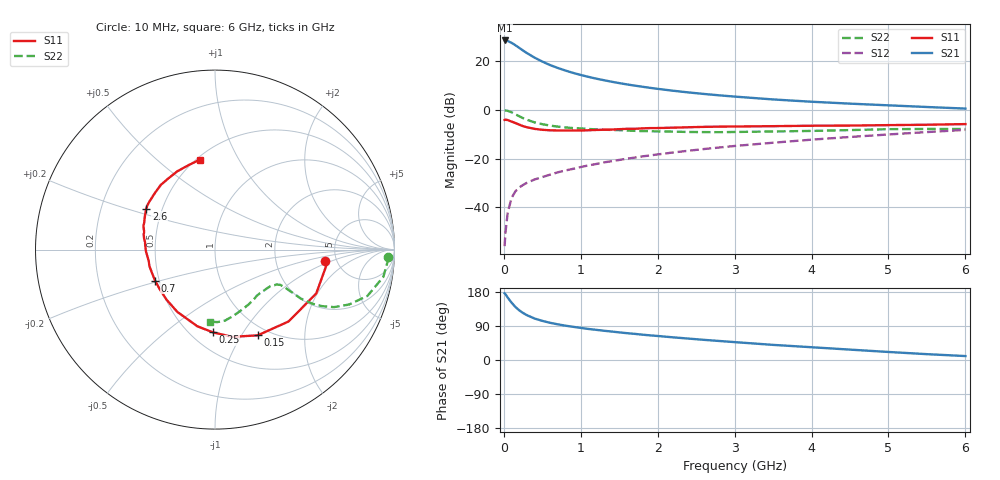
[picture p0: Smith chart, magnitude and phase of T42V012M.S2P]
! Infineon Technologies  Discrete & RF Semiconductors
! BFR182T
! Si NPN RF Bipolar Junction Transistor in SC75
! VCE = 2 V  IC = 12 mA
! Common Emitter S-Parameters:  October  1999
# GHz  S  MA  R  50
!  f  S11  S21  S12  S22
! GHz  MAG  ANG  MAG  ANG  MAG  ANG  MAG  ANG
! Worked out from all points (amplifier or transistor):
!   36 points, 10 MHz to 6 GHz, reference 50 ohm
!   highest |S21| = 28.4 dB at 10 MHz (marker M1)
!   |S21| within 3 dB of that: start of sweep to 198.7 MHz
!   unconditionally stable (mu >= 1): 825.6 MHz to 3.767 GHz
!   at 250 MHz: K = 0.52, MSG = 27.5 dB, |S12| = -30.8 dB
!   at 1.4 GHz: K = 1.10, MAG = 14.3 dB, |S12| = -21.1 dB
!   at 6 GHz: K = 0.84, MSG = 4.4 dB, |S12| = -8.3 dB
!   S11 on the Smith chart (normalised r, x): 10 MHz: 4.07, -0.82; 150 MHz: 0.88, -1.18; 250 MHz: 0.64, -0.74; 700 MHz: 0.47, -0.19; 2.6 GHz: 0.41, +0.23; 6 GHz: 0.52, +0.70
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0.01  0.6188 -5.8  26.3 176.0  0.0016 72.8  0.9661 -2.5
0.02  0.6265 -8.2  26.28 174.0  0.0029 91.9  0.9655 -3.6
0.05  0.6148 -23.4  25.65 164.8  0.0077 82.0  0.9501 -9.2
0.1  0.5732 -44.3  23.52 151.5  0.0156 72.2  0.8878 -16.9
0.15  0.5337 -63.5  21 140.0  0.0212 66.7  0.8068 -22.3
0.2  0.4956 -78.9  18.56 131.1  0.0255 63.8  0.7364 -25.8
0.25  0.4608 -91.6  16.34 124.0  0.0288 60.1  0.6726 -27.9
0.3  0.4383 -103.0  14.48 118.3  0.0318 59.6  0.6237 -29.0
0.4  0.4055 -121.2  11.68 109.4  0.0373 58.5  0.55 -29.7
0.5  0.3884 -134.0  9.708 103.3  0.0417 59.9  0.506 -29.2
0.6  0.3789 -144.4  8.25 98.2  0.0467 60.4  0.4741 -28.9
0.7  0.376 -152.7  7.192 94.2  0.0521 62.0  0.4507 -28.5
0.9  0.3767 -165.8  5.693 87.6  0.0615 64.6  0.4208 -28.4
1.1  0.3799 -175.3  4.717 81.9  0.0723 65.6  0.404 -29.0
1.3  0.3892 176.8  4.033 77.2  0.0833 66.4  0.3896 -30.2
1.6  0.4064 167.9  3.305 70.8  0.0994 67.2  0.3744 -32.5
2.2  0.4293 156.0  2.453 59.8  0.133 67.8  0.356 -39.7
2.6  0.4458 149.2  2.108 53.2  0.1565 67.0  0.3482 -45.2
3.5  0.4605 136.3  1.626 39.9  0.2109 64.3  0.3586 -58.6
4.5  0.4739 123.5  1.334 27.4  0.2767 59.4  0.3829 -74.4
5.5  0.4929 107.5  1.138 15.4  0.3486 53.4  0.4041 -88.0
6  0.5081 99.6  1.056 10.4  0.3868 49.6  0.4027 -93.6
